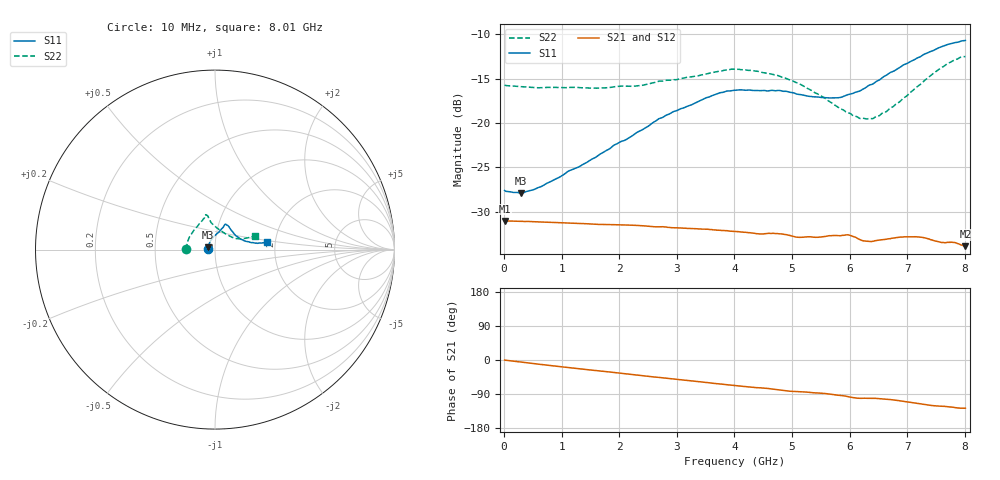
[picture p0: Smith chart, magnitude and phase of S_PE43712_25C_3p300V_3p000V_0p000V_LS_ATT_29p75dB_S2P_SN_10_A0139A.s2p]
! DEVICE ID: PE43712
! File Path: z:\PE43713\PE43713_CHAR_NOM_04292014\AMB\3p300\LS_ATT_29p75dB\PE43713_AMB_3p300V_3p000V_0p000V_LS_ATT_29p75dB_S2P_SN_10_A0139A.s2p
! Serial: 10
! Lot: A0139A
! Temp: 25C
! VDD: 3.300
! VSS: 0.000
! Control_Hi: 3.000
! Control_Lo: 0.000
! Attenuation Step: 29.75dB
! Port 1: RF1
! Port 2: RF2
! ThroughPath:1-2
! IDD: 0.0001459862
! ISS: -6.97e-008
#  Hz  S  RI  R  50
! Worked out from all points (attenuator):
!   801 points, 10 MHz to 8.01 GHz, reference 50 ohm
!   highest |S21| = -31.03 dB at 10 MHz (marker M1); lowest = -33.9 dB at 8.01 GHz (marker M2)
!   lowest |S11| = -27.9 dB at 290 MHz (marker M3), VSWR 1.08, Z = 46.3 + j1.23 ohm
!   |S11| at or under -10 dB: start of sweep to end of sweep
!   |S22| runs from -19.5 to -12.5 dB; largest |S21 - S12| = 0.0001
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1e7  -0.0416 0.000906  0.0281 -0.000125  0.0281 -0.000131  -0.1633 0.00114
2.9e8  -0.0381 0.0133  0.0278 -0.00265  0.0278 -0.00265  -0.1592 0.0184
6.5e8  -0.0338 0.0281  0.0271 -0.0057  0.0271 -0.00569  -0.153 0.0393
1.35e9  -0.021 0.054  0.0248 -0.011  0.0248 -0.011  -0.1379 0.0771
2.28e9  0.0095 0.0868  0.0205 -0.0168  0.0205 -0.0168  -0.102 0.125
2.68e9  0.025 0.1023  0.0181 -0.0187  0.0181 -0.0187  -0.0833 0.1503
3.5e9  0.0484 0.1297  0.0129 -0.0216  0.0129 -0.0217  -0.0574 0.1796
3.74e9  0.0533 0.1379  0.0113 -0.0222  0.0113 -0.0222  -0.0543 0.1884
4.01e9  0.0582 0.1415  0.00943 -0.0226  0.0094 -0.0226  -0.0526 0.194
4.31e9  0.0617 0.1396  0.00745 -0.0228  0.00746 -0.0228  -0.0462 0.1922
4.76e9  0.0721 0.1345  0.00468 -0.0233  0.00472 -0.0233  -0.0369 0.1812
5.09e9  0.082 0.1201  0.00266 -0.0226  0.00267 -0.0226  -0.0289 0.1659
5.35e9  0.0911 0.1073  0.00153 -0.0228  0.0015 -0.0227  -0.0215 0.1504
5.82e9  0.1143 0.0792  -0.00134 -0.0231  -0.00131 -0.0232  0.00991 0.1209
5.99e9  0.1269 0.0704  -0.00297 -0.0232  -0.00293 -0.0232  0.025 0.1111
6.18e9  0.1394 0.0595  -0.00423 -0.0216  -0.00416 -0.0216  0.0437 0.0967
6.4e9  0.1574 0.0521  -0.00409 -0.0211  -0.00406 -0.0212  0.067 0.0819
6.68e9  0.1852 0.0435  -0.00539 -0.0216  -0.00541 -0.0216  0.0985 0.0674
7.15e9  0.2272 0.0361  -0.00922 -0.0209  -0.00918 -0.0209  0.1459 0.0607
7.56e9  0.2637 0.0376  -0.0112 -0.0182  -0.0112 -0.0182  0.1902 0.0675
7.81e9  0.2801 0.0407  -0.0122 -0.0174  -0.0122 -0.0174  0.2134 0.0744
8.01e9  0.2886 0.0433  -0.0122 -0.0161  -0.0122 -0.0161  0.2243 0.0763
